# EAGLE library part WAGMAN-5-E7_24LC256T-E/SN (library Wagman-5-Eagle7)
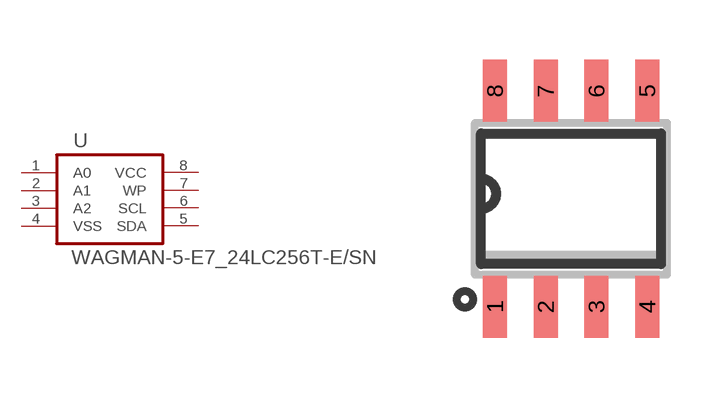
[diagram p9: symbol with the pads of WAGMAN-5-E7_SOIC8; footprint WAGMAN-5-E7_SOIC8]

Designator prefix U

## WAGMAN-5-E7_24LC256T-E/SN  [WAGMAN-5-E7_SOIC8]
1  A0  pwr
2  A1  pas
3  A2  pas
4  VSS  pas
5  SDA  pas
6  SCL  pas
7  WP  pas
8  VCC  pas

## Footprint WAGMAN-5-E7_SOIC8 (pad centres in mm)
Small Outline IC
smd 0.6 x 1.55: 1 -1.905,-2.7; 2 -0.635,-2.7; 3 0.635,-2.7; 4 1.905,-2.7; 5 1.905,2.7; 6 0.635,2.7; 7 -0.635,2.7; 8 -1.905,2.7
